PROGRAM p07_pomnilnaCelica
VAR
	S0: BOOL;
	S1: BOOL;
	L0: BOOL;
	L1: BOOL;
	L2: BOOL;
	RS_celica: RS;
	SR_celica: SR;
END_VAR

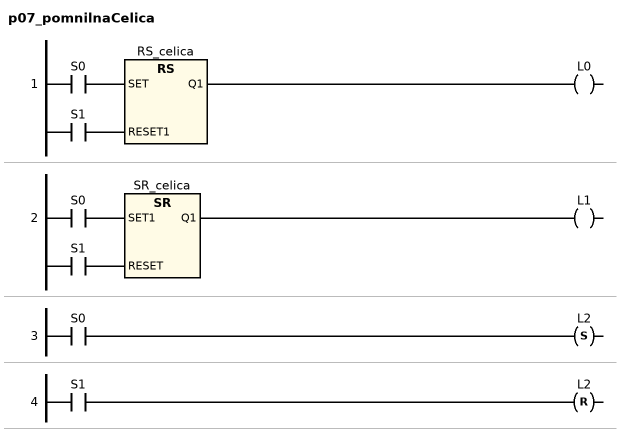
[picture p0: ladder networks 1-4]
// NETWORK 1
RS_celica(SET := S0, RESET1 := S1); // RS
L0 := RS_celica.Q1;

// NETWORK 2
SR_celica(SET1 := S0, RESET := S1); // SR
L1 := SR_celica.Q1;

// NETWORK 3
L2 S= S0;

// NETWORK 4
L2 R= S1;

END_PROGRAM
